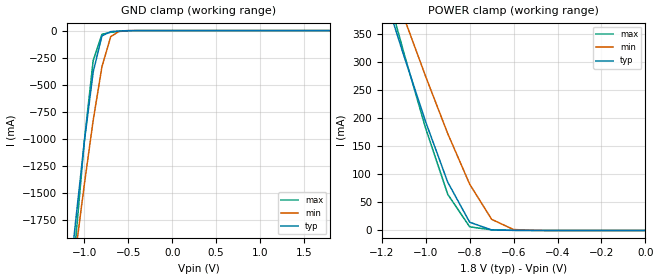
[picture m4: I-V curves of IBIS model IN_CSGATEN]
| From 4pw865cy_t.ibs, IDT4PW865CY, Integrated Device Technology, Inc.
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|   Model IN_CSGATEN
[Model]   IN_CSGATEN
Model_type   Input
Vinl =  0.000V
Vinh =  1.80000V
C_comp   3.00000pF   3.0000pF   3.00000pF
[Temperature Range]   25.00000   0.11000k   0.000
[Voltage Range]   1.80000V   1.70000V   1.90000V
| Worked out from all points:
|   GND clamp passes 1 mA (typ) near -0.51 V on its own axis
|   POWER clamp passes 1 mA (typ) near -0.70 V on its own axis
[GND_clamp]
| voltage   I(typ)   I(min)   I(max)
-1.8V     -7.509A    -6.777A    -9.219A
-1.2V     -2.552A    -2.699A    -2.933A
-1.1V     -1.768A    -2.049A    -1.943A
-1V       -1.025A    -1.42A     -1.018A
-900mV    -384.3mA   -831.8mA   -278.9mA
-800mV    -49.16mA   -334.1mA   -34.6mA
-700mV    -9.52mA    -55.82mA   -15.97mA
-600mV    -3.358mA   -4.767mA   -7.725mA
-400mV    -53.67uA   -34.09uA   -242.5uA
1.8V      26.95pA    5.248nA    -19.88pA
[POWER_clamp]
| voltage   I(typ)   I(min)   I(max)
-1.8V     1.209A     1.169A     1.353A
-1.2V     434.4mA    488.7mA    458.3mA
-1.1V     311.1mA    379.5mA    316.3mA
-1V       192.7mA    273.3mA    181mA
-900mV    85.9mA     172.3mA    64.37mA
-800mV    14.67mA    82.28mA    6.452mA
-700mV    926.3uA    19.77mA    1.156mA
-600mV    137.1uA    1.636mA    359.6uA
-500mV    21.08uA    107.7uA    70.28uA
0V        26.95pA    124.4pA    8.257pA
